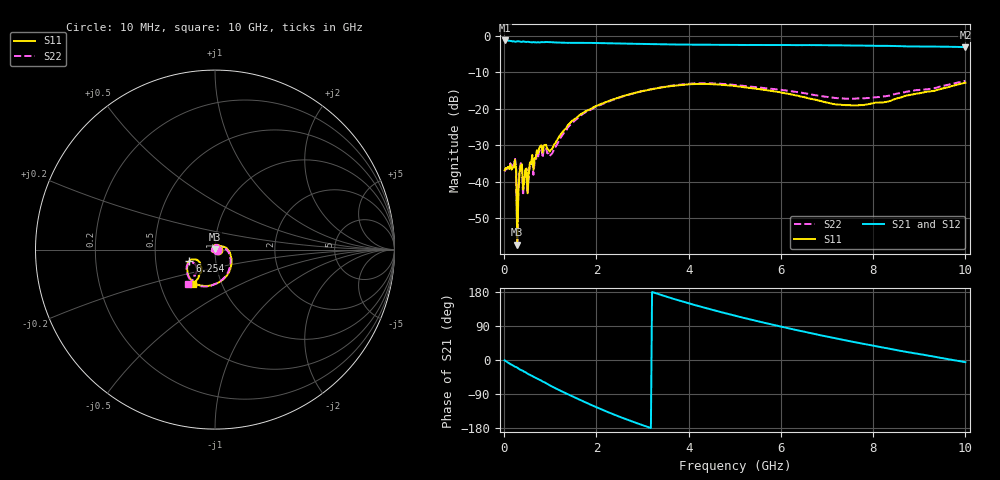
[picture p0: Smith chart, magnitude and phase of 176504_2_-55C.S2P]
!  2-Port S-parameters saved by WinCal
! VAR MeasName=S-Parameters (CALIBRATED_DATA) read from VNA (N5242A)
! VAR MeasDate=2017-11-2 17:07:43
! VAR NAME=176504_2_-55C
! VAR FILENAME=176504_2_-55C.S2P
! VAR DATE=2017-11-2 17:07:43
! VAR PHYS_PORTS=2,3
# Hz S DB R 50
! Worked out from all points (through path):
!   401 points, 10 MHz to 10 GHz, reference 50 ohm
!   highest |S21| = -1.29 dB at 10 MHz (marker M1); lowest = -3.1 dB at 10 GHz (marker M2)
!   lowest |S11| = -57.3 dB at 284.7 MHz (marker M3), VSWR 1.00, Z = 50 + j0.132 ohm
!   |S11| at or under -10 dB: start of sweep to end of sweep
!   |S22| runs from -57.7 to -12.4 dB; largest |S21 - S12| = 0.0068
!   S11 on the Smith chart (normalised r, x): 10 MHz: 1.03, -0.00; 6.254 GHz: 0.75, -0.10; 10 GHz: 0.73, -0.29
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1e7  -36.86 -4.1  -1.29 -0.9  -1.29 -1.0  -37.27 -3.0
2.098e8  -36.19 -122.5  -1.51 -16.0  -1.51 -16.0  -35.56 -123.5
2.34775e8  -34.05 -151.5  -1.62 -17.7  -1.62 -17.7  -33.53 -150.8
2.84725e8  -57.31 104.4  -1.49 -20.2  -1.49 -20.2  -57.74 162.8
3.34675e8  -37.55 -147.6  -1.58 -24.6  -1.58 -24.6  -36.71 -145.1
3.5965e8  -35.59 -170.9  -1.65 -26.2  -1.65 -26.2  -34.97 -167.4
3.84625e8  -35.26 156.2  -1.70 -27.4  -1.70 -27.4  -35.07 160.8
4.34575e8  -40.23 -174.6  -1.61 -31.2  -1.62 -31.2  -39.41 -165.5
4.5955e8  -36.64 108.1  -1.66 -31.9  -1.66 -31.9  -37.47 112.8
7.5925e8  -30.82 77.3  -1.83 -51.7  -1.83 -51.7  -31.76 79.0
9.84025e8  -31.81 30.1  -1.73 -66.6  -1.73 -66.5  -33.09 23.4
1.433575e9  -23.86 7.6  -1.95 -93.3  -1.94 -93.3  -24.43 4.6
1.683325e9  -21.37 -13.0  -1.94 -107.3  -1.94 -107.3  -21.67 -16.2
2.482525e9  -16.94 -54.7  -2.11 -148.9  -2.10 -148.8  -17.06 -56.9
3.35665e9  -14.32 -89.8  -2.33 173.5  -2.34 173.5  -14.25 -91.0
4.180825e9  -13.21 -117.1  -2.47 143.4  -2.49 143.6  -13.05 -116.0
5.005e9  -13.78 -137.0  -2.51 116.9  -2.51 117.1  -13.51 -134.8
6.25375e9  -16.17 -156.3  -2.55 81.2  -2.56 81.5  -15.26 -151.7
6.678325e9  -17.39 -156.2  -2.56 70.1  -2.58 70.2  -16.15 -152.0
7.55245e9  -19.08 -141.6  -2.68 48.1  -2.68 48.2  -17.25 -142.8
8.35165e9  -17.94 -126.0  -2.77 29.6  -2.80 29.8  -16.43 -131.1
1e10  -12.87 -122.9  -3.11 -5.7  -3.13 -5.3  -12.37 -127.9
